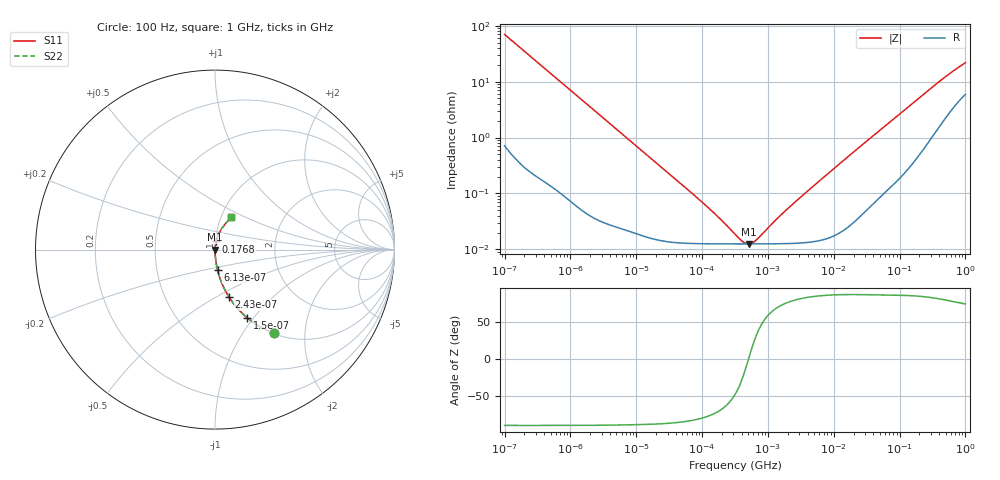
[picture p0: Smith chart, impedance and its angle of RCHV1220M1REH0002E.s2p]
! RCHV1220M1REH0002E  S-PARAMETER MODEL  (AEC-Q200 qualified)
! Model Generated by ELNA Corporation (http://www.ty-top.com)
! Version 1.0
! ELNA Control No. 240229
! Copyright (c) 2024 ELNA CO.,LTD. All Rights Reserved.
! Products Name : CONDUCTIVE POLYMER HYBRID ALUMINUM ELECTROLYTIC CAPACITORS
! Characteristics :
!  Capacitance  :  22uF  ,  Rated voltage  :  80V
!  Operating Temp. Range  :  -55 to +105 degC  ,  Endurance  :  10000hr at 105 degC
!  Dimension D  :  8mm  ,  Dimension L  :  10mm
! Frequency Range : 100Hz - 1GHz
! External Node Assignments :
!  1  o---| |---o  2
# MHz S RI R 50
!Freq[MHz].  S11 Real  S11 Imag  S21 Real  S21 Imag  S12 Real  S12 Imag  S22 Real  S22 Imag
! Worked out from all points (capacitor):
!   401 points, 100 Hz to 1 GHz, reference 50 ohm
!   read as one part in series: C = 22.9 uF near 108 Hz
!   lowest |Z| = 12.5 mohm at 512.9 kHz (marker M1)
!   series resonance near 507.7 kHz, so ESL is about 4.3 nH
!   S11 on the Smith chart (normalised r, x): 100 Hz: 1.01, -1.39; 150 Hz: 1.01, -0.93; 243 Hz: 1.00, -0.57; 613 Hz: 1.00, -0.23; 176.8 MHz: 1.01, +0.09; 1 GHz: 1.12, +0.42
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0.0001  0.3282 -0.4645  0.6718 0.4645  0.6718 0.4645  0.3282 -0.4645
0.00015  0.1803 -0.3801  0.8197 0.3801  0.8197 0.3801  0.1803 -0.3801
0.000243  0.0782 -0.2643  0.9218 0.2643  0.9218 0.2643  0.0782 -0.2643
0.000378  0.0345 -0.1781  0.9655 0.1781  0.9655 0.1781  0.0345 -0.1781
0.000613  0.014 -0.1125  0.986 0.1125  0.986 0.1125  0.014 -0.1125
0.001488  0.00273 -0.0472  0.9973 0.0472  0.9973 0.0472  0.00273 -0.0472
0.004241  0.000544 -0.0167  0.9995 0.0167  0.9995 0.0167  0.000544 -0.0167
0.022131  0.000156 -0.00323  0.9998 0.00323  0.9998 0.00323  0.000156 -0.00323
0.12517  0.000126 -0.000538  0.9999 0.000538  0.9999 0.000538  0.000126 -0.000538
0.203002  0.000126 -0.000297  0.9999 0.000297  0.9999 0.000297  0.000126 -0.000297
0.316228  0.000125 -0.000139  0.9999 0.000139  0.9999 0.000139  0.000125 -0.000139
0.419276  0.000125 -5.44e-05  0.9999 5.44e-05  0.9999 5.44e-05  0.000125 -5.44e-05
0.512861  0.000125 2.88e-06  0.9999 -2.88e-06  0.9999 -2.88e-06  0.000125 2.88e-06
0.578762  0.000125 3.71e-05  0.9999 -3.71e-05  0.9999 -3.71e-05  0.000125 3.71e-05
0.679986  0.000126 8.37e-05  0.9999 -8.37e-05  0.9999 -8.37e-05  0.000126 8.37e-05
1.650061  0.000127 0.000416  0.9999 -0.000416  0.9999 -0.000416  0.000127 0.000416
4.704354  0.000138 0.00129  0.9999 -0.00129  0.9999 -0.00129  0.000138 0.00129
69.9842  0.00157 0.0185  0.9984 -0.0185  0.9984 -0.0185  0.00157 0.0185
176.8072  0.00608 0.0452  0.9939 -0.0452  0.9939 -0.0452  0.00608 0.0452
504.0806  0.0357 0.1145  0.9643 -0.1145  0.9643 -0.1145  0.0357 0.1145
785.2356  0.0681 0.156  0.9319 -0.156  0.9319 -0.156  0.0681 0.156
1000  0.0913 0.1796  0.9087 -0.1796  0.9087 -0.1796  0.0913 0.1796
